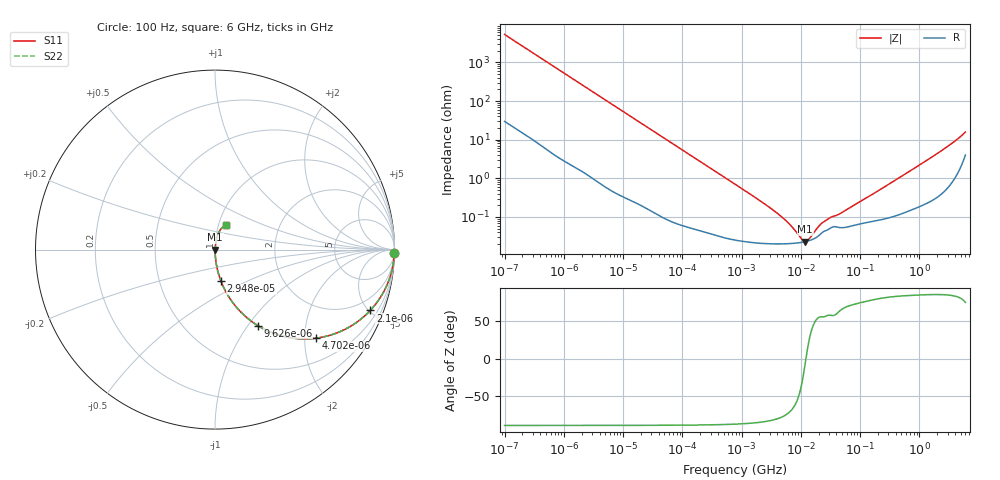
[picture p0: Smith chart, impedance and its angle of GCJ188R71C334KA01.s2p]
!Murata Part Number: GCJ188R71C334KA01
!These Parameters are Measured in Series Mode Connection
!Data Generated on Mar 13, 2026
!  o--ll--o
!Port1  Port2
!  o------o
!Operation Temp=25[degC], DC Bias Voltage=0[V]
!Freq. Start=100[Hz] Stop=6[GHz] 401[Steps]
# Hz S RI R 50
!Freq.(Hz) S11(Real) S11(Imag) S21(Real) S21(Imag) S12(Real) S12(Imag) S22(Real) S22(Imag)
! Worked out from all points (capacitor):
!   401 points, 100 Hz to 6 GHz, reference 50 ohm
!   read as one part in series: C = 301 nF near 109 Hz
!   lowest |Z| = 23.1 mohm at 11.89 MHz (marker M1)
!   series resonance near 12.22 MHz, so ESL is about 560 pH
!   S11 on the Smith chart (normalised r, x): 100 Hz: open; 2.1 kHz: 1.03, -5.09; 4.702 kHz: 1.01, -2.28; 9.626 kHz: 1.01, -1.12; 29.48 kHz: 1.00, -0.37; 6 GHz: 1.08, +0.30
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100  0.9995 -0.0189  0.000464 0.0189  0.000464 0.0189  0.9995 -0.0189
600  0.9869 -0.1111  0.0131 0.1111  0.0131 0.1111  0.9869 -0.1111
2008  0.8748 -0.3281  0.1252 0.3281  0.1252 0.3281  0.8748 -0.3281
2100  0.8648 -0.3391  0.1352 0.3391  0.1352 0.3391  0.8648 -0.3391
4702  0.5646 -0.493  0.4354 0.493  0.4354 0.493  0.5646 -0.493
9626  0.2387 -0.4233  0.7613 0.4233  0.7613 0.4233  0.2387 -0.4233
15752  0.1062 -0.3046  0.8938 0.3046  0.8938 0.3046  0.1062 -0.3046
29482  0.0337 -0.1766  0.9663 0.1766  0.9663 0.1766  0.0337 -0.1766
40335  0.0187 -0.1313  0.9813 0.1313  0.9813 0.1313  0.0187 -0.1313
129199  0.00229 -0.0419  0.9977 0.0419  0.9977 0.0419  0.00229 -0.0419
774597  0.000302 -0.00706  0.9997 0.00706  0.9997 0.00706  0.000302 -0.00706
4246196  0.000202 -0.00115  0.9998 0.00115  0.9998 0.00115  0.000202 -0.00115
6644369  0.000205 -0.000587  0.9998 0.000587  0.9998 0.000587  0.000205 -0.000587
1.039699e7  0.000221 -0.000147  0.9998 0.000147  0.9998 0.000147  0.000221 -0.000147
1.189169e7  0.000229 -2.42e-05  0.9998 2.42e-05  0.9998 2.42e-05  0.000229 -2.42e-05
1.555665e7  0.00026 0.000223  0.9997 -0.000223  0.9997 -0.000223  0.00026 0.000223
2.035112e7  0.000334 0.000483  0.9997 -0.000483  0.9997 -0.000483  0.000334 0.000483
2.545746e7  0.000434 0.000649  0.9996 -0.000649  0.9996 -0.000649  0.000434 0.000649
4.764863e7  0.000529 0.00114  0.9995 -0.00114  0.9995 -0.00114  0.000529 0.00114
3.124326e8  0.001 0.00711  0.999 -0.00711  0.999 -0.00711  0.001 0.00711
1.95892e9  0.00493 0.0423  0.9951 -0.0423  0.9951 -0.0423  0.00493 0.0423
6e9  0.0586 0.1378  0.9414 -0.1378  0.9414 -0.1378  0.0586 0.1378
